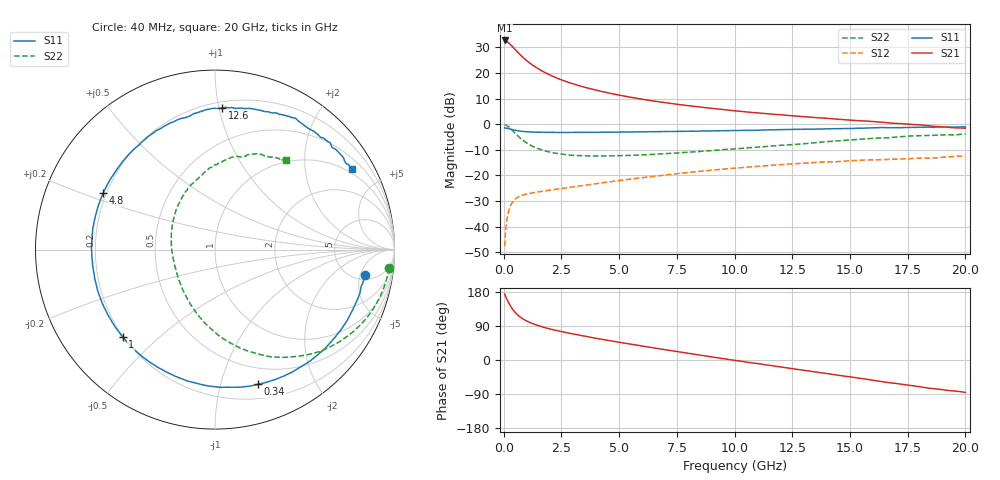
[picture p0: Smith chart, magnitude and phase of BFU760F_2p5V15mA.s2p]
! Filename:  P:\Prog\Test\Noise\ATS_data\Testdata_Net\Split files Spar\BFU760F_2W_C1_Bias4_2.5V_5mA_30mA_D.s2p
! Date/Time: Mon 06/Feb/2012 15:08:14
! BFU760_2W_C1_Bias4_2.5V_5mA_30mA_R.s2p
! MDIF S-parameter v. bias file
! BFU760_2W_C1_2.5V_5mA_30mA
! Date/time Fri Mar 18 11:16:19 2011
! VAR V_out= 2.5000
! VAR I_out= 14.9600
! VAR V_in= 0.7784
! VAR I_in= 0.0438
! Device data file deembeded for feedlines and parallel
! Original file: \Split files Spar\BFU760_2W_C1_Bias4_2.5V_5mA_30mA_R.s2p
! Feed-files: PR003V01_101208_Feed1.s2p, PR003V01_101208_Feed2.s2p
! Parallel-file: PR003V01_101208_Par.s2p
# MHz S MA R 50
!  Freq-MHz  S11-mag  S11-arg  S21-mag  S21-arg  S12-mag  S12-arg  S22-mag  S22-arg
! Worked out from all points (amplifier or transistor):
!   167 points, 40 MHz to 20 GHz, reference 50 ohm
!   highest |S21| = 32.7 dB at 40 MHz (marker M1)
!   |S21| within 3 dB of that: start of sweep to 442.5 MHz
!   unconditionally stable (mu >= 1): 4.686 GHz to 13.53 GHz
!   at 550 MHz: K = 0.20, MSG = 28.8 dB, |S12| = -28.9 dB
!   at 4.2 GHz: K = 0.96, MSG = 17.9 dB, |S12| = -23.0 dB
!   at 20 GHz: K = 0.86, MSG = 5.5 dB, |S12| = -12.5 dB
!   S11 on the Smith chart (normalised r, x): 40 MHz: 6.04, -5.94; 340 MHz: 0.33, -1.32; 1 GHz: 0.20, -0.38; 4.8 GHz: 0.19, +0.23; 12.6 GHz: 0.24, +1.02; 20 GHz: 0.85, +3.48
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40  0.8458 -9.5  43 174.2  0.004139 75.1  0.9737 -6.1
50  0.8448 -12.5  42.91 172.3  0.004721 74.8  0.9715 -7.9
120  0.8353 -28.2  41.52 163.0  0.01185 73.2  0.9472 -18.9
180  0.8245 -41.5  39.73 155.4  0.01716 67.8  0.9096 -27.8
240  0.8093 -54.0  37.83 148.2  0.02176 62.7  0.8654 -36.1
340  0.788 -72.2  34.01 138.1  0.02785 55.0  0.7823 -48.4
400  0.7744 -82.2  31.99 132.8  0.03073 51.2  0.7328 -54.6
480  0.7601 -93.2  29.11 126.8  0.03379 46.8  0.6747 -62.4
650  0.7334 -112.0  24.14 116.5  0.03817 40.3  0.5666 -75.6
800  0.7209 -124.4  20.73 109.7  0.04083 36.5  0.497 -84.9
1000  0.708 -136.7  17.26 102.8  0.04326 33.6  0.4283 -95.3
1400  0.6959 -153.5  12.8 92.7  0.0468 30.8  0.3448 -111.6
1950  0.6875 -168.1  9.346 82.7  0.05091 30.0  0.2879 -128.3
2500  0.6879 -178.2  7.314 75.0  0.05509 30.5  0.261 -141.9
3400  0.6903 169.2  5.415 64.1  0.06299 30.8  0.242 -158.3
4800  0.6979 153.3  3.835 48.8  0.077 30.0  0.2409 -179.0
6800  0.7127 134.5  2.697 29.0  0.09927 25.1  0.2617 157.9
10200  0.7532 106.2  1.787 -2.6  0.1401 10.0  0.3354 125.3
12600  0.7895 87.2  1.442 -23.8  0.1687 -3.4  0.4007 105.2
13400  0.795 81.5  1.353 -30.6  0.1776 -8.9  0.4288 98.7
16800  0.8529 55.3  1.046 -60.3  0.2056 -30.2  0.547 72.0
20000  0.8837 30.4  0.8327 -85.6  0.2358 -52.0  0.6388 51.7
